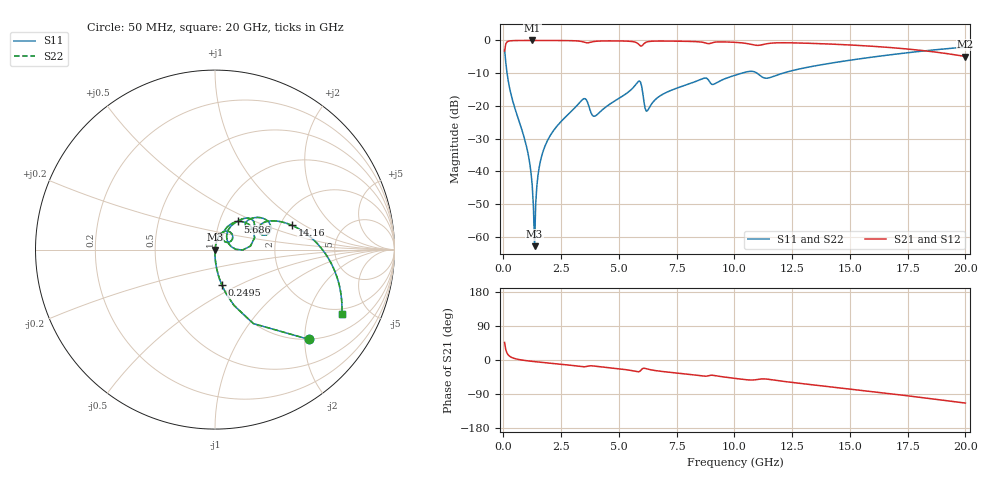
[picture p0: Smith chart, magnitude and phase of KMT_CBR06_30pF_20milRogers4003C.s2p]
! Data measured by Modelithics Inc. support@modelithics.com 813-866-6335
! KEMET CBR0603 30pF, Pad Width= 0.851mm, Pad Length= 0.64mm, Pad Gap= 0.62mm, 20mil Rogers 4003C substrate Data, January 2022
# hz S ma R 50
! 2 Port Network Data from SP1.SP block
! freq  magS11  angS11  magS21  angS21  magS12  angS12  magS22  angS22
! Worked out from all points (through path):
!   401 points, 50 MHz to 20 GHz, reference 50 ohm
!   highest |S21| = -0.01 dB at 1.247 GHz (marker M1); lowest = -4.9 dB at 20 GHz (marker M2)
!   group delay of S21, straight-line fit = 15.8 ps
!   lowest |S11| = -62.9 dB at 1.347 GHz (marker M3), VSWR 1.00, Z = 50.1 + j0.0141 ohm
!   |S11| at or under -10 dB: 156.6 MHz to 10.32 GHz (10.16 GHz wide, 194 % of centre); 10.98 GHz to 12.1 GHz (1.122 GHz wide, 9.72 % of centre)
!   |S22| runs from -62.9 to -2.0 dB; largest |S21 - S12| = 0
!   S11 on the Smith chart (normalised r, x): 50 MHz: 1.00, -2.10; 249.5 MHz: 1.00, -0.41; 5.686 GHz: 1.22, +0.40; 14.16 GHz: 2.31, +0.78; 20 GHz: 1.75, -3.34
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5e7  0.7248 -43.7  0.6885 46.3  0.6885 46.3  0.7248 -43.7
2.495e8  0.1999 -79.1  0.9794 10.7  0.9794 10.7  0.1999 -79.1
1.0475e9  0.02 -90.5  0.9992 -2.2  0.9992 -2.2  0.02 -90.5
1.14725e9  0.01266 -90.1  0.9992 -2.9  0.9992 -2.9  0.01266 -90.1
1.247e9  0.006006 -87.3  0.9993 -3.6  0.9993 -3.6  0.006006 -87.3
1.34675e9  0.0007187 11.3  0.9993 -4.3  0.9993 -4.3  0.0007187 11.3
1.4465e9  0.006004 78.1  0.9992 -4.9  0.9992 -4.9  0.006004 78.1
1.496375e9  0.008755 79.9  0.9992 -5.3  0.9992 -5.3  0.008755 79.9
1.596125e9  0.01408 80.9  0.9991 -5.9  0.9991 -5.9  0.01408 80.9
1.8455e9  0.02659 80.7  0.9987 -7.4  0.9987 -7.4  0.02659 80.7
3.391625e9  0.1219 57.9  0.9623 -17.5  0.9623 -17.5  0.1219 57.9
3.990125e9  0.07063 50.4  0.9699 -16.4  0.9699 -16.4  0.07063 50.4
5.685875e9  0.2029 50.6  0.9448 -29.5  0.9448 -29.5  0.2029 50.6
5.885375e9  0.2405 27.9  0.8525 -30.4  0.8525 -30.4  0.2405 27.9
6.2345e9  0.08441 35.1  0.9537 -23.9  0.9537 -23.9  0.08441 35.1
6.73325e9  0.1385 56.1  0.9788 -29.2  0.9788 -29.2  0.1385 56.1
1.0025e10  0.2939 37.6  0.9356 -48.5  0.9356 -48.5  0.2939 37.6
1.14215e10  0.2651 23.3  0.8927 -50.5  0.8927 -50.5  0.2651 23.3
1.336662e10  0.4012 22.7  0.9013 -65.3  0.9013 -65.3  0.4012 22.7
1.416462e10  0.4489 17.6  0.8798 -70.7  0.8798 -70.7  0.4489 17.6
1.670825e10  0.6011 -0.3  0.7806 -88.6  0.7806 -88.6  0.6011 -0.3
2e10  0.7916 -26.8  0.5681 -113.7  0.5681 -113.7  0.7916 -26.8
